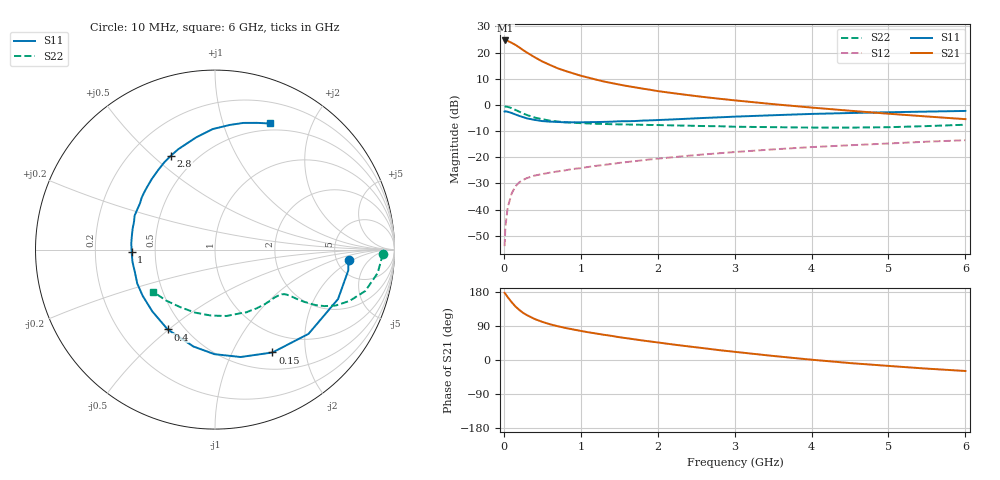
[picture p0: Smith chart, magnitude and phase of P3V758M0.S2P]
! SIEMENS Small Signal Semiconductors
! BFP181
! Si NPN RF Bipolar Junction Transistor in SOT143
! VCE = 0.75 V  IC = 8 mA
! Common Emitter S-Parameters:  March  1996
# GHz  S  MA  R  50
!  f  S11  S21  S12  S22
! GHz  MAG  ANG  MAG  ANG  MAG  ANG  MAG  ANG
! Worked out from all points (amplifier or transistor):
!   36 points, 10 MHz to 6 GHz, reference 50 ohm
!   highest |S21| = 24.6 dB at 20 MHz (marker M1)
!   |S21| within 3 dB of that: start of sweep to 217.8 MHz
!   unconditionally stable (mu >= 1): 632.8 MHz to end of sweep
!   at 250 MHz: K = 0.48, MSG = 24.8 dB, |S12| = -28.7 dB
!   at 1.4 GHz: K = 1.52, MAG = 11.2 dB, |S12| = -22.6 dB
!   at 6 GHz: K = 1.43, MAG = 0.1 dB, |S12| = -13.5 dB
!   S11 on the Smith chart (normalised r, x): 10 MHz: 6.40, -1.73; 150 MHz: 0.72, -1.45; 400 MHz: 0.41, -0.50; 1 GHz: 0.37, -0.01; 2.8 GHz: 0.36, +0.57; 6 GHz: 0.42, +1.44
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0.01  0.7463 -4.6  16.98 177.2  0.002 82.6  0.9355 -1.5
0.02  0.7515 -8.9  17.01 174.7  0.0047 84.5  0.9291 -3.2
0.05  0.7388 -21.9  16.64 165.9  0.0109 79.5  0.9156 -8.2
0.1  0.7014 -42.0  15.38 153.0  0.02 69.1  0.8685 -15.4
0.15  0.6566 -60.8  14.01 141.4  0.0278 61.0  0.8022 -20.9
0.2  0.6152 -76.6  12.57 132.3  0.0331 54.6  0.7422 -24.8
0.25  0.5826 -90.3  11.14 124.4  0.0368 50.1  0.6865 -27.3
0.3  0.5532 -102.5  9.989 118.4  0.04 46.6  0.6402 -28.9
0.4  0.517 -120.7  8.137 108.2  0.0446 43.4  0.5733 -30.4
0.5  0.4903 -135.5  6.75 100.6  0.0477 40.9  0.5307 -31.1
0.6  0.4782 -147.4  5.787 94.3  0.0508 41.0  0.5012 -31.5
0.7  0.4726 -156.4  4.996 89.2  0.0536 40.5  0.4805 -31.9
0.8  0.4634 -164.8  4.447 84.6  0.0563 40.3  0.4665 -32.3
1  0.4645 -178.4  3.608 76.7  0.0619 41.1  0.4479 -33.8
1.1  0.4678 175.6  3.31 73.1  0.0653 41.2  0.4413 -34.8
1.5  0.4864 157.1  2.445 60.2  0.0779 42.3  0.4243 -39.5
2.2  0.5278 131.9  1.675 40.9  0.1001 40.8  0.4053 -51.3
2.8  0.5783 115.1  1.311 26.0  0.1192 37.8  0.3908 -63.4
3.5  0.6341 99.5  1.033 10.7  0.1412 33.4  0.3753 -80.1
4.5  0.6992 83.3  0.773 -8.1  0.1694 25.6  0.3681 -107.3
5.5  0.7441 71.6  0.6 -22.8  0.1982 18.3  0.3936 -133.9
6  0.7663 66.5  0.534 -29.0  0.2114 14.0  0.4178 -146.0
